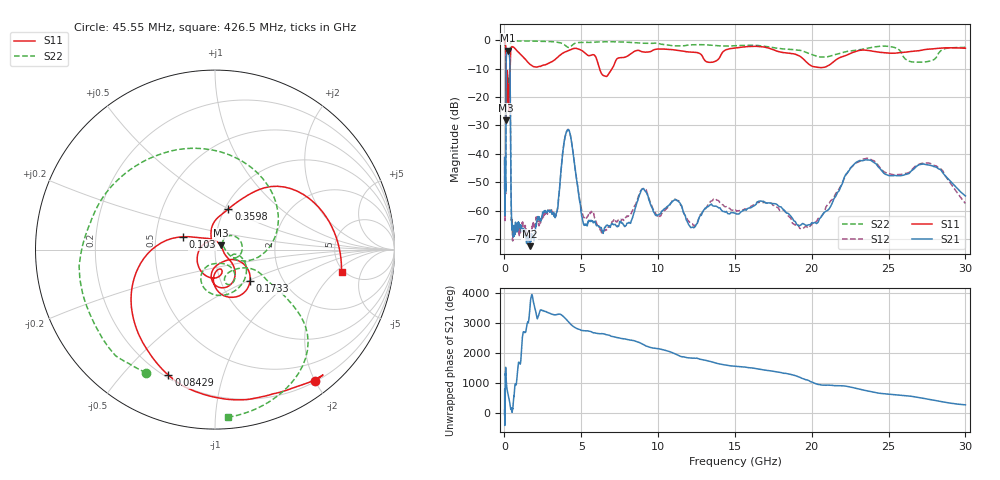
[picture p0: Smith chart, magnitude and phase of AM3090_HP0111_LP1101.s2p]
! Date/Time: Thu, Feb 28, 2019 2:01 PM
! Network Analyzer: Agilent Technologies E8364B Rev: A.07.50.67
! Sweep from 0.010 to 30.000 GHz, 1601 Points, Sweep Type: LOG
! Power Supply: 5.023 V, 0.002 A
# Hz S DB R 50
!freq MagS11 AngS11 MagS21 AngS21 MagS12 AngS12 MagS22 AngS22
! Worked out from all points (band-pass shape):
!   1601 points, 10 MHz to 30 GHz, reference 50 ohm
!   highest |S21| = -3.66 dB at 243.5 MHz (marker M1); lowest = -72.6 dB at 1.639 GHz (marker M2)
!   |S21| within 3 dB of the highest: 115.9 MHz to 344.3 MHz (228.4 MHz wide, 99.3 % of centre)
!   lowest |S11| = -28.3 dB at 109.9 MHz (marker M3), VSWR 1.08, Z = 53.1 + j2.47 ohm
!   |S11| at or under -10 dB: 100.6 MHz to 370.4 MHz (269.8 MHz wide, 115 % of centre); 6.184 GHz to 7.009 GHz (824.8 MHz wide, 12.5 % of centre)
!   |S22| runs from -25.9 to -0.1 dB; largest |S21 - S12| = 0.01
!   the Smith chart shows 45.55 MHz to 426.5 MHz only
!   S11 on the Smith chart (normalised r, x): 45.55 MHz: 0.21, -2.01; 84.29 MHz: 0.21, -0.67; 103 MHz: 0.69, +0.10; 173.3 MHz: 1.37, -0.52; 359.8 MHz: 1.04, +0.50; 426.5 MHz: 4.72, -2.46
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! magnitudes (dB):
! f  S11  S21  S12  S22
! 10 MHz  -0.3  -41.3  -42.1  -0.7
! 38.04 MHz  -0.5  -61.3  -61.5  -1.6
! 45.55 MHz  -0.7  -52.5  -55.0  -2.1
! 84.29 MHz  -2.5  -51.3  -53.2  -4.6
! 103 MHz  -14.4  -15.5  -15.5  -13.9
! 109.9 MHz  -28.3  -8.7  -8.7  -25.5
! 144.7 MHz  -21.4  -4.2  -4.2  -19.5
! 173.3 MHz  -11.6  -3.8  -3.8  -13.5
! 243.5 MHz  -18.7  -3.7  -3.6  -20.9
! 359.8 MHz  -12.4  -9.3  -9.2  -8.2
! 426.5 MHz  -2.9  -52.7  -53.7  -0.6
! 550.5 MHz  -2.4  -65.5  -69.2  -0.2
! 1.639 GHz  -8.4  -72.6  -69.0  -0.3
! 2.084 GHz  -9.5  -64.3  -62.6  -0.3
! 3.352 GHz  -6.5  -61.9  -62.0  -0.7
! 4.136 GHz  -3.8  -31.5  -31.4  -2.5
! 5.18 GHz  -4.2  -65.1  -62.5  -0.8
! 7.926 GHz  -5.8  -65.2  -62.3  -0.7
! 9.027 GHz  -4.1  -52.2  -52.3  -1.1
! 19.51 GHz  -6.9  -64.8  -66.0  -4.0
! 23.48 GHz  -3.5  -42.2  -41.8  -3.0
! 30 GHz  -2.9  -54.9  -57.5  -2.5
